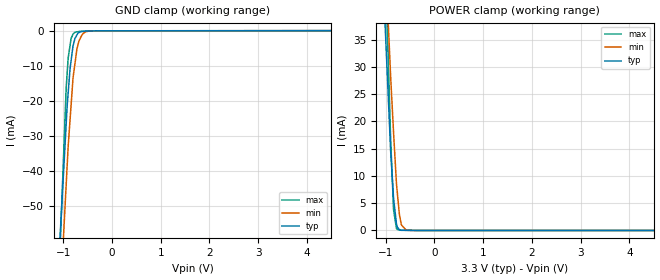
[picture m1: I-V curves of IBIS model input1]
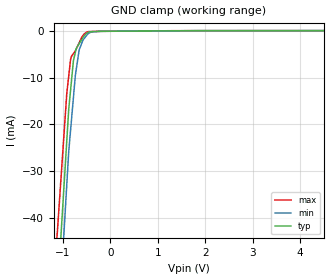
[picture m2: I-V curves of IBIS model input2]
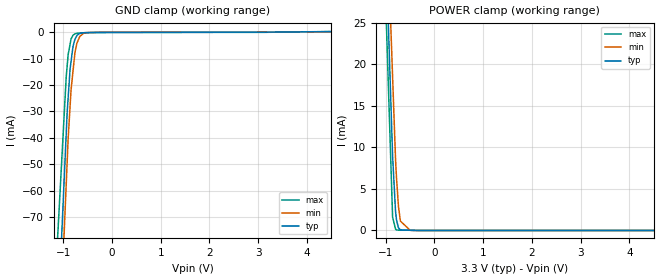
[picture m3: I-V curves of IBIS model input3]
| Teraspeed (R) Labs.
| http://www.teraspeed.com
[IBIS Ver]   3.2
[Comment Char] |_char
[File Name]   dac5672a.ibs
[File Rev]   3.1
[Source]  Teraspeed (R) Labs.
[Date]   10-12-2006
[Notes]   Quality Check of this IBIS model: Model Passes IBIS Check
   Model parses into ICX IS. Simulation done with Hyperlynx.
   1. MIN TYP MAX information is based on Temprature and Voltage
   characteristics only.
[Disclaimer]
| Use: Teraspeed (R) Labs has licensed Teraspeed (R) AccuModel (tm)
| IBIS models to specific integrated circuit suppliers ("IC Vendors")
| for use and distribution as  follows: Each IC Vendor may use IBIS
| Models, and distribute them to IC Vendor's customers to use solely
| for developing printed circuit board designs. Users of this model may
| modify the IBIS model to suit its specific applications but
| rights to derivative works and such modifications shell belong
| to Teraspeed (R) Labs. No other distribution of these materials is
| permitted.
| DISCLAIMER OF WARRANTY: UNLESS OTHERWISE AGREED TO IN WRITING
| TERASPEED (R) LABS DISCLAIMS AND USER WAIVES ALL WARRANTIES,
| EXPRESS OR IMPLIED, INCLUDING WARRANTIES OF MERCHANTABILITY AND
| FITNESS FOR A PARTICULAR PURPOSE. IN NO EVENT SHALL
| TERASPEED BE LIABLE FOR ANY DIRECT OR INDIRECT DAMAGES,
| WHETHER IN CONTRACT OR TORT, INCLUDING, WITHOUT LIMITATION,
| LOST PROFITS, BUSINESS INTERRUPTION, OR LOST INFORMATION
| ARISING OUT OF THE USE OF OR THE INABILITY TO USE THE MODEL,
| EVEN IF TERASPEED (R) Labs HAS BEEN ADVISED OF THE POSSIBILITY
| OF SUCH DAMAGES.
[Copyright]
| This file is the legal property of Teraspeed (R) Labs Copyright(c) 2006.
| All other rights are reserved.
[Component]   DAC5672A
[Manufacturer] TI
[Package]
| variable   typ   min   max
R_pkg  1.6023E-02  1.6023E-02  1.6023E-02
L_pkg  2.2032E-09  2.2032E-09  2.2032E-09
C_pkg  7.2832E-13  7.2832E-13  7.2832E-13
[Pin] signal_name  model_name  R_pin  L_pin C_pin
1   DA13   input1   1.80E-02   1.76E-09   4.16E-13
2   DA12   input1   1.72E-02   1.68E-09   3.97E-13
3   DA11   input1   1.64E-02   1.60E-09   3.78E-13
4   DA10   input1   1.56E-02   1.52E-09   3.60E-13
5   DA9   input1   1.49E-02   1.45E-09   3.43E-13
6   DA8   input1   1.41E-02   1.38E-09   3.26E-13
7   DA7   input1   1.41E-02   1.38E-09   3.26E-13
8   DA6   input1   1.49E-02   1.45E-09   3.43E-13
9   DA5   input1   1.56E-02   1.52E-09   3.60E-13
10   DA4   input1   1.64E-02   1.60E-09   3.78E-13
11   DA3   input1   1.72E-02   1.68E-09   3.97E-13
12   DA2   input1   1.80E-02   1.76E-09   4.16E-13
13   DA1   input1   1.80E-02   1.76E-09   4.16E-13
14   DA0   input1   1.72E-02   1.68E-09   3.97E-13
15   DGND   GND   1.64E-02   1.60E-09   3.78E-13
16   DVDD   POWER   1.56E-02   1.52E-09   3.60E-13
17   WRTA/IQ   input1   1.49E-02   1.45E-09   3.43E-13
18   CLKA/IQ   input1   1.41E-02   1.38E-09   3.26E-13
19   CLKB/RESIQ input1   1.41E-02   1.38E-09   3.26E-13
20   WRTB/SELIQ input1   1.49E-02   1.45E-09   3.43E-13
21   DGND   GND   1.56E-02   1.52E-09   3.60E-13
22   DVDD   POWER   1.64E-02   1.60E-09   3.78E-13
23   DB13   input1   1.72E-02   1.68E-09   3.97E-13
24   DB12   input1   1.80E-02   1.76E-09   4.16E-13
25   DB11   input1   1.80E-02   1.76E-09   4.16E-13
26   DB10   input1   1.72E-02   1.68E-09   3.97E-13
27   DB9   input1   1.64E-02   1.60E-09   3.78E-13
28   DB8   input1   1.56E-02   1.52E-09   3.60E-13
29   DB7   input1   1.49E-02   1.45E-09   3.43E-13
30   DB6   input1   1.41E-02   1.38E-09   3.26E-13
31   DB5   input1   1.41E-02   1.38E-09   3.26E-13
32   DB4   input1   1.49E-02   1.45E-09   3.43E-13
33   DB3   input1   1.56E-02   1.52E-09   3.60E-13
34   DB2   input1   1.64E-02   1.60E-09   3.78E-13
35   DB1   input1   1.72E-02   1.68E-09   3.97E-13
36   DB0   input1   1.80E-02   1.76E-09   4.16E-13
37   SLEEP   input1   1.80E-02   1.76E-09   4.16E-13
38   AGND   GND   1.72E-02   1.68E-09   3.97E-13
39   IOUTB1   term   1.64E-02   1.60E-09   3.78E-13
40   IOUTB2   term   1.56E-02   1.52E-09   3.60E-13
41   BIASJ_B   term   1.49E-02   1.45E-09   3.43E-13
42   GSET   input2   1.41E-02   1.38E-09   3.26E-13
43   EXTIO   term   1.41E-02   1.38E-09   3.26E-13
44   BIASJ_A   term   1.49E-02   1.45E-09   3.43E-13
45   IOUTA2   term   1.56E-02   1.52E-09   3.60E-13
46   IOUTA1   term   1.64E-02   1.60E-09   3.78E-13
47   AVDD   POWER   1.72E-02   1.68E-09   3.97E-13
48   MODE   input3   1.80E-02   1.76E-09   4.16E-13
[Diff Pin] inv_pin vdiff tdelay_typ tdelay_min tdelay_max
39  40   NA  NA  NA  NA
46  45   NA  NA  NA  NA
[Model] term
Model_type Terminator
C_comp  0.00000pF 0.00000pF 0.00000pF
[Voltage Range] 3.30000V 3.00000V 3.60000V
| Models and submodels in the file (4): term (Terminator), input1 (Input), input2 (Input), input3 (Input)
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[Model] input1
Model_type Input
Vinl = 800.000mV
Vinh = 2.00000V
C_comp 830.000fF 830.000fF 830.000fF
| variable typ   min   max
[Voltage Range] 3.30000V 3.00000V 3.60000V
[POWER Clamp Reference] 3.30000V 3.00000V 3.60000V
[GND Clamp Reference] 0.00000V 0.00000V 0.00000V
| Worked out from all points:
|   GND clamp passes 1 mA (typ) near -0.71 V on its own axis
|   POWER clamp passes 1 mA (typ) near -0.77 V on its own axis
[GND Clamp]
-3.3V     -632.2mA   -680.7mA   -876.1mA
-940mV    -26.61mA   -43.95mA   -16.32mA
-900mV    -17.89mA   -33.16mA   -7.858mA
-860mV    -10.72mA   -25.31mA   -4.103mA
-840mV    -8.599mA   -21.39mA   -2.225mA
-800mV    -4.357mA   -13.54mA   -945.7uA
-760mV    -2.19mA    -9.379mA   -476.6uA
-720mV    -1.213mA   -5.218mA   -307.3uA
-680mV    -542.8uA   -2.982mA   -227.4uA
-580mV    -150.5uA   -644.4uA   -145.3uA
-480mV    -66.45uA   -106.1uA   -92.49uA
6.6V      39.79uA    45.89uA    51.35uA
[POWER Clamp]
-3.3V     502.7mA    509.8mA    725.7mA
-1.04V    43.04mA    56.28mA    58.09mA
-900mV    14.57mA    28.18mA    16.74mA
-840mV    5.866mA    17.91mA    3.806mA
-780mV    1.145mA    8.507mA    360.2uA
-760mV    578.6uA    6.634mA    208.1uA
-720mV    133uA      2.889mA    53.84uA
-680mV    27.72uA    1.038mA    49.53uA
-580mV    19.57uA    47.66uA    38.76uA
6.6V      0A         0A         0A
[Model] input2
Model_type Input
Vinl = 800.000mV
Vinh = 2.00000V
C_comp 830.000fF 830.000fF 830.000fF
| variable typ   min   max
[Voltage Range] 3.30000V 3.00000V 3.60000V
[POWER Clamp Reference] 3.30000V 3.00000V 3.60000V
[GND Clamp Reference] 0.00000V 0.00000V 0.00000V
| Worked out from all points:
|   GND clamp passes 1 mA (typ) near -0.54 V on its own axis
[GND Clamp]
-3.3V     -415.1mA   -445.5mA   -366.5mA
-920mV    -23.42mA   -32.77mA   -13.33mA
-880mV    -16.84mA   -25.83mA   -9.72mA
-840mV    -12.65mA   -21.18mA   -6.11mA
-780mV    -6.368mA   -14.21mA   -4.888mA
-740mV    -4.64mA    -9.561mA   -4.321mA
-660mV    -2.796mA   -4.137mA   -2.607mA
-580mV    -1.49mA    -2.008mA   -1.043mA
-500mV    -531.5uA   -996.8uA   -315.5uA
-400mV    -201.6uA   -273uA     -186uA
-200mV    -137.3uA   -141uA     -137.7uA
6.6V      18.03uA    16.41uA    19.64uA
[POWER Clamp]
-3.3V     0A         0A         0A
6.6V      0A         0A         0A
[Model] input3
Model_type Input
Vinl = 800.000mV
Vinh = 2.00000V
C_comp 830.000fF 830.000fF 830.000fF
| variable typ   min   max
[Voltage Range] 3.30000V 3.00000V 3.60000V
[POWER Clamp Reference] 3.30000V 3.00000V 3.60000V
[GND Clamp Reference] 0.00000V 0.00000V 0.00000V
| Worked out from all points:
|   GND clamp passes 1 mA (typ) near -0.70 V on its own axis
|   POWER clamp passes 1 mA (typ) near -0.77 V on its own axis
[GND Clamp]
-3.3V     -1.018A    -1.087A    -831.7mA
-940mV    -38.69mA   -57.82mA   -17.06mA
-920mV    -30.39mA   -49.1mA    -12.8mA
-900mV    -24.89mA   -40.38mA   -8.537mA
-860mV    -13.9mA    -28.03mA   -4.558mA
-840mV    -11.07mA   -21.85mA   -2.569mA
-800mV    -5.41mA    -14.75mA   -1.164mA
-760mV    -2.685mA   -7.658mA   -638.2uA
-720mV    -1.301mA   -4.196mA   -451.4uA
-660mV    -523.2uA   -1.599mA   -327.5uA
-520mV    -175uA     -177.1uA   -252.9uA
6.6V      573.3uA    359.6uA    609.9uA
[POWER Clamp]
-3.3V     451.4mA    420.1mA    505.3mA
-1.08V    48.87mA    54.71mA    41.75mA
-860mV    8.976mA    18.5mA     1.604mA
-800mV    2.339mA    8.623mA    185.3uA
-780mV    1.275mA    6.369mA    52.41uA
-740mV    322.5uA    2.918mA    48.53uA
-700mV    69.25uA    1.131mA    44.65uA
-500mV    29.68uA    21.47uA    25.24uA
6.6V      0A         0A         0A
